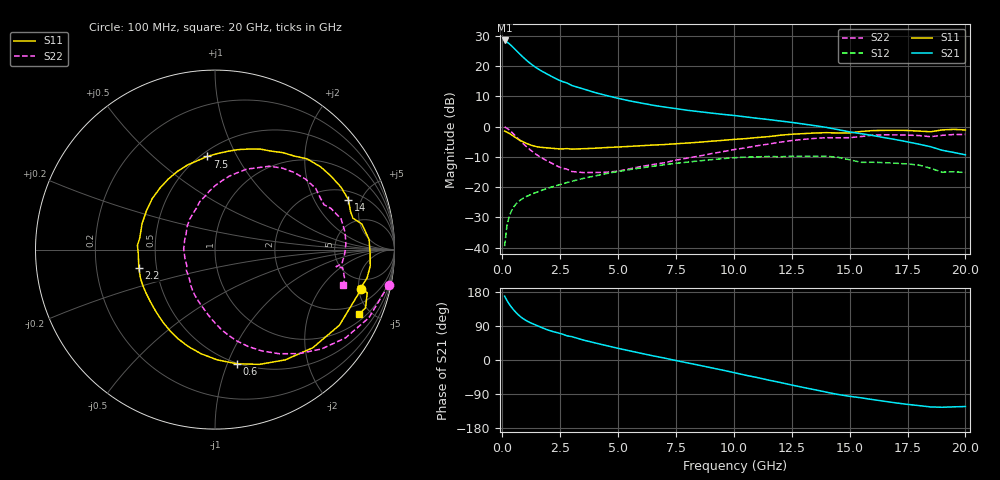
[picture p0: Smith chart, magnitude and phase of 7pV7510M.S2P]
! Infineon Technologies  Discrete & RF Semiconductors
! bfp620
! VCE = 0.75 V,  IC =  10 mA
! Common Emitter S-Parameters:  Sep 2002
# GHz  S  MA  R  50
!  f  S11  S21  S12  S22
! GHz  MAG  ANG  MAG  ANG  MAG  ANG  MAG  ANG
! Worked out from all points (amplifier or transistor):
!   59 points, 100 MHz to 20 GHz, reference 50 ohm
!   highest |S21| = 28.5 dB at 100 MHz (marker M1)
!   |S21| within 3 dB of that: start of sweep to 561.3 MHz
!   unconditionally stable (mu >= 1): 4.1 GHz to 10.52 GHz; 16.96 GHz to end of sweep
!   at 1 GHz: K = 0.50, MSG = 22.7 dB, |S12| = -23.2 dB
!   at 5.5 GHz: K = 1.05, MAG = 10.0 dB, |S12| = -14.2 dB
!   at 20 GHz: K = 1.51, MAG = -1.3 dB, |S12| = -15.2 dB
!   S11 on the Smith chart (normalised r, x): 100 MHz: 3.51, -5.35; 600 MHz: 0.49, -1.08; 2.2 GHz: 0.40, -0.10; 7.5 GHz: 0.54, +0.76; 14 GHz: 2.58, +3.89; 20 GHz: 1.36, -4.30
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0.1  0.8446 -15.0  26.46 168.5  0.0106 79.6  0.9875 -11.5
0.2  0.8112 -31.3  25 157.0  0.0231 74.0  0.9377 -23.9
0.3  0.7719 -45.1  23.33 147.4  0.033 68.3  0.8778 -34.1
0.4  0.7285 -57.5  21.55 139.0  0.0409 63.0  0.8117 -43.0
0.5  0.6859 -68.8  19.78 131.5  0.0475 58.6  0.7447 -51.1
0.6  0.6474 -79.3  18.11 124.9  0.0531 54.8  0.681 -58.4
0.8  0.5851 -97.7  15.21 113.7  0.062 49.4  0.5705 -71.1
0.9  0.5599 -105.5  13.99 109.1  0.0656 47.5  0.5242 -76.4
1.1  0.5179 -118.8  11.96 101.8  0.0718 44.8  0.4471 -85.4
1.3  0.4861 -129.8  10.4 96.0  0.0774 43.1  0.387 -92.9
1.6  0.4584 -144.0  8.706 88.3  0.0856 41.3  0.3216 -103.5
2.2  0.4367 -166.4  6.528 74.8  0.1022 38.3  0.241 -124.0
3  0.4242 171.2  4.784 61.7  0.1249 33.8  0.1815 -149.6
3.5  0.4315 160.3  4.182 52.6  0.1395 30.4  0.1741 -164.7
5  0.4602 131.7  2.931 30.8  0.1816 18.7  0.1837 151.1
7  0.5053 101.1  2.106 5.1  0.2345 1.3  0.253 114.1
7.5  0.5209 94.8  1.982 -1.4  0.248 -3.7  0.2796 107.8
10.5  0.6329 60.0  1.449 -40.1  0.3131 -36.2  0.4466 73.7
13.5  0.7834 26.4  1.036 -78.5  0.3233 -69.8  0.6387 38.1
14  0.7939 20.5  0.97 -84.9  0.3237 -76.4  0.6567 31.4
17  0.8696 -6.0  0.609 -113.2  0.2481 -100.4  0.7298 2.4
20  0.8799 -24.0  0.342 -122.8  0.1745 -112.5  0.7422 -15.4
